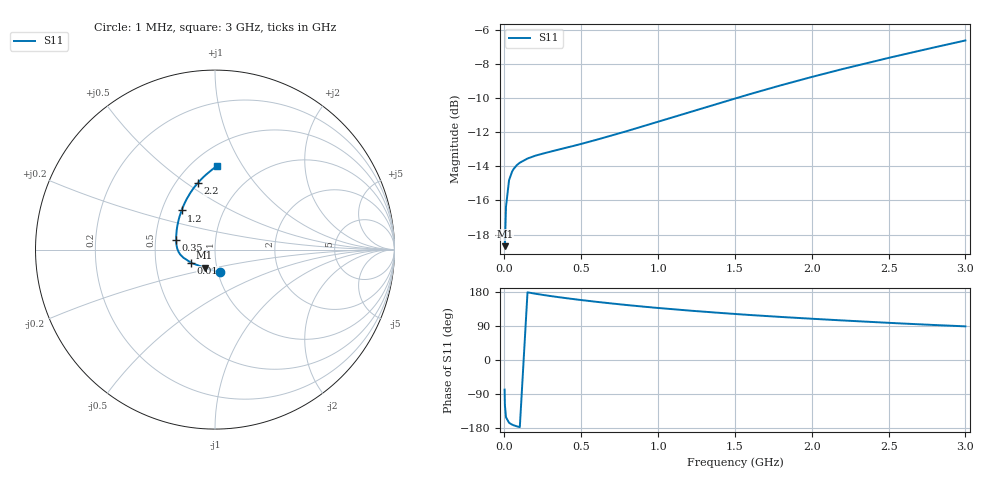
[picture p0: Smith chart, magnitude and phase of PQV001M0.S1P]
! SIEMENS Small Signal Semiconductors
! BAR64-04
! Si PIN Diode in SOT23 (2 diodes in series, pin 3 open)
! IF = 1 mA
! S-Parameters:  July  1992
# GHz  S  MA  R  50
!  f  S11
! GHz  MAG  ANG
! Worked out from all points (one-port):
!   33 points, 1 MHz to 3 GHz, reference 50 ohm
!   lowest |S11| = -18.7 dB at 3 MHz (marker M1), VSWR 1.26, Z = 43.7 - j8.96 ohm
!   |S11| at or under -10 dB: start of sweep to 1.515 GHz
!   S11 on the Smith chart (normalised r, x): 1 MHz: 1.02, -0.26; 10 MHz: 0.76, -0.11; 350 MHz: 0.64, +0.07; 1.2 GHz: 0.63, +0.30; 2.2 GHz: 0.64, +0.56; 3 GHz: 0.65, +0.78
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0.001  0.1299 -78.1
0.003  0.1165 -119.7
0.01  0.152 -151.1
0.03  0.1818 -165.7
0.05  0.1926 -170.6
0.06  0.196 -172.3
0.08  0.201 -175.0
0.1  0.2044 -177.1
0.15  0.2102 178.6
0.2  0.2142 175.0
0.25  0.2173 171.8
0.35  0.2231 166.0
0.4  0.226 163.3
0.5  0.232 158.2
0.6  0.2386 153.5
0.7  0.2457 149.1
0.8  0.2531 144.9
1  0.2694 137.3
1.2  0.2867 130.5
1.4  0.3051 124.4
1.6  0.3246 118.7
1.8  0.3443 113.6
2  0.3641 108.9
2.2  0.384 104.4
2.4  0.4037 100.2
2.5  0.414 98.1
2.8  0.4446 92.3
3  0.4656 88.8
